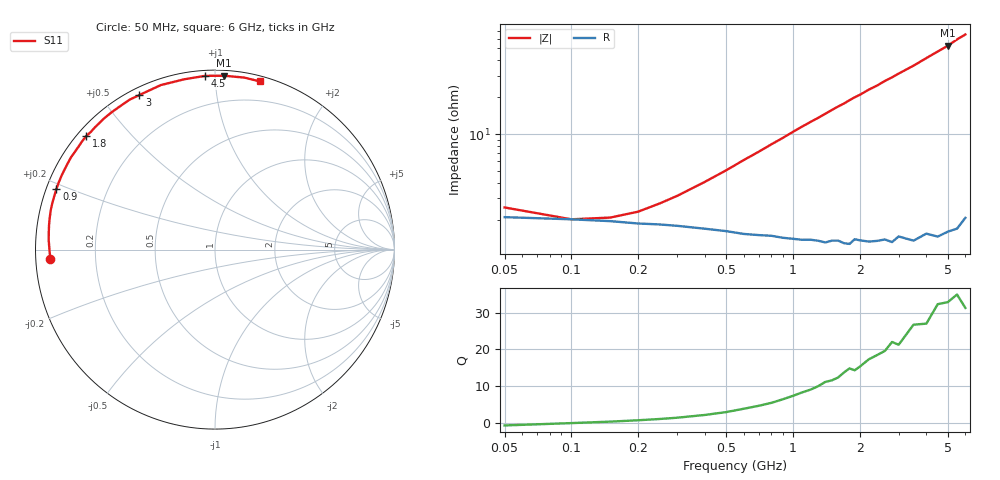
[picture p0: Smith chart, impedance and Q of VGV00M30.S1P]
! Infineon Technologies  Discrete & RF Semiconductors
! BB 831
! Si Tuning Diode in SOD323
! VR =
! S-Parameters:  July  1999
# GHz  S  MA  R  50
!  f  S11
! GHz  MAG  ANG
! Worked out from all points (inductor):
!   34 points, 50 MHz to 6 GHz, reference 50 ohm
!   read as one part to ground: L = 1.62 nH near 600 MHz
!   highest Q = 32.9 at 5 GHz (marker M1), where L = 1.68 nH
!   S11 on the Smith chart (normalised r, x): 50 MHz: 0.04, -0.03; 900 MHz: 0.03, +0.18; 1.8 GHz: 0.03, +0.38; 3 GHz: 0.03, +0.62; 4.5 GHz: 0.03, +0.94; 6 GHz: 0.04, +1.30
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0.05  0.9193 -176.8
0.1  0.9223 -179.9
0.15  0.9249 178.3
0.2  0.928 176.8
0.4  0.9348 171.5
0.5  0.9379 169.0
0.6  0.9412 166.4
0.8  0.9438 161.5
0.9  0.9462 159.1
1.1  0.949 154.2
1.2  0.9494 151.9
1.4  0.9529 147.4
1.6  0.9525 142.9
1.7  0.9552 140.9
1.8  0.9564 138.6
1.9  0.9532 136.5
2  0.9546 134.7
2.2  0.957 130.5
2.4  0.9577 127.0
2.6  0.9581 123.0
2.8  0.9613 119.7
3  0.9587 116.1
3.5  0.9651 108.2
4  0.9642 100.3
4.5  0.9696 93.3
5  0.9701 87.0
5.5  0.9722 80.3
6  0.9696 75.1
